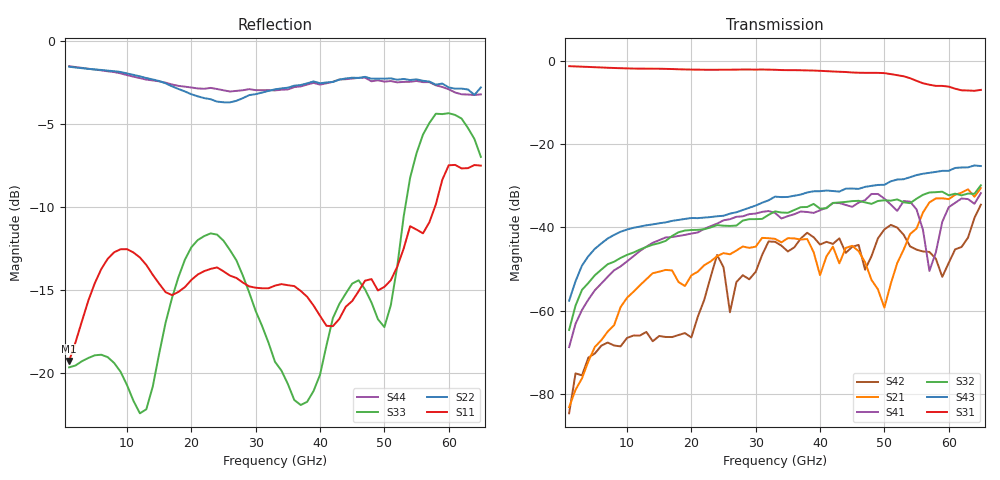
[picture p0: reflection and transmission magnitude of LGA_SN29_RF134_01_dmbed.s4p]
! Created Thu Nov 10 13:44:36 2022
# hz S ma R 50
! 4 Port Network Data from SP1.SP block
! freq  magS11  angS11  magS12  angS12  magS13  angS13  magS14  angS14
!  magS21  angS21  magS22  angS22  magS23  angS23  magS24  angS24
!  magS31  angS31  magS32  angS32  magS33  angS33  magS34  angS34
!  magS41  angS41  magS42  angS42  magS43  angS43  magS44  angS44
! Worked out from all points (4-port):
!   65 points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, 1 GHz to 65 GHz, reference 50 ohm
!   strongest paths, dB at 1 GHz, 17 GHz, 33 GHz, 49 GHz, 65 GHz:
!     S31: -1.3, -2.0, -2.2, -2.9, -7.0
!     S43: -57.6, -38.4, -32.6, -29.8, -25.3
!     S32: -64.6, -42.1, -36.2, -33.7, -29.9
!     S41: -68.7, -42.3, -36.5, -32.0, -31.8
!     S21: -83.2, -50.3, -42.8, -54.9, -30.6
!     S42: -84.6, -66.3, -43.5, -42.6, -34.6
!   lowest |S11| = -19.3 dB at 1 GHz (marker M1), VSWR 1.24, Z = 60.4 - j6.01 ohm
!   |S11| at or under -10 dB: start of sweep to 57.85 GHz
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1e9  0.109 -26.8  9.181e-05 -129.4  0.8601 -13.7  0.0003249 -108.0
     6.948e-05 125.7  0.8361 171.1  0.0006046 65.6  0.0001536 69.3
     0.8591 -13.7  0.0005874 71.9  0.1042 -26.0  0.001162 78.3
     0.0003658 -115.5  5.872e-05 42.2  0.001318 72.2  0.8392 171.3
1.9e10  0.1818 173.4  0.001893 -32.0  0.786 115.2  0.008232 -25.0
        0.001979 -29.0  0.7044 2.7  0.009253 -155.7  0.0006282 -162.4
        0.785 115.3  0.00916 -156.0  0.2198 153.8  0.01265 -125.1
        0.008124 -25.2  0.0005387 -150.7  0.01262 -125.5  0.7283 2.9
2.8e10  0.1875 64.0  0.005581 -162.6  0.7839 -0.3  0.01355 -142.8
        0.005891 -161.5  0.6723 -101.1  0.01226 97.4  0.002988 73.9
        0.783 -0.3  0.01207 98.1  0.1969 62.2  0.01618 131.1
        0.01357 -145.2  0.002666 67.6  0.01615 130.8  0.7103 -101.7
3.5e10  0.1841 -71.3  0.007664 96.1  0.7701 -93.6  0.01346 118.3
        0.00742 98.4  0.723 176.5  0.01541 20.6  0.005364 -13.1
        0.7698 -93.6  0.01496 22.5  0.0929 7.1  0.02317 52.1
        0.01364 118.9  0.005139 -13.9  0.02315 52.2  0.7143 -172.7
5e10  0.182 -166.1  0.0003888 91.0  0.7095 55.6  0.02277 -67.1
      0.001088 93.5  0.7694 47.8  0.02118 -168.3  0.00922 -147.6
      0.7091 56.1  0.02114 -168.3  0.1377 66.1  0.0329 -97.4
      0.02213 -67.3  0.009445 -150.2  0.03239 -97.3  0.754 47.8
5.7e10  0.2849 177.2  0.02032 5.4  0.5153 -46.9  0.00268 86.8
        0.01993 12.2  0.7544 -21.3  0.02539 102.7  0.006051 87.0
        0.5145 -46.3  0.02622 103.4  0.5663 -93.2  0.04464 167.1
        0.002999 86.4  0.005071 79.6  0.04513 166.3  0.7513 -18.2
6.5e10  0.4215 134.4  0.02939 -120.0  0.4459 -150.0  0.0276 -148.0
        0.02964 -118.6  0.7244 -131.9  0.03166 9.0  0.01824 163.2
        0.4462 -149.5  0.03196 13.4  0.4476 -159.4  0.05515 45.8
        0.02577 -150.5  0.01871 172.2  0.05443 45.7  0.6903 -126.6
